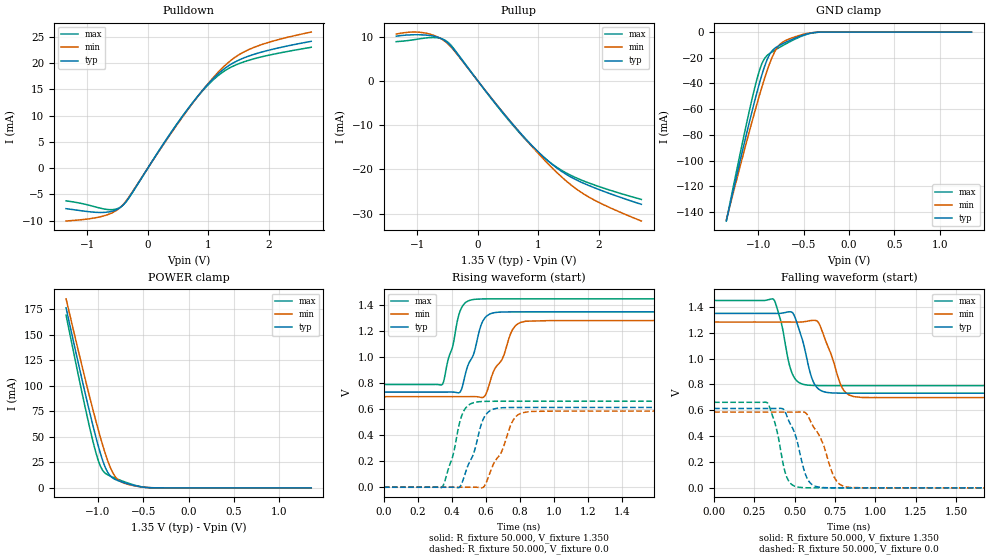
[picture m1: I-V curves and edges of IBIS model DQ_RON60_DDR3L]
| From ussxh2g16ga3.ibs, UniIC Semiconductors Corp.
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|   Model DQ_RON60_DDR3L
[Model] DQ_RON60_DDR3L
Model_type I/O
Vinl =  0.540V
Vinh =  0.810V
Vmeas =  0.675V
Rref =  50.000
Vref =  0.675V
C_comp   0.966pF   0.965pF   0.967pF
[Model Spec]
Vinh   0.810V   0.776V   0.860V
Vinl   0.540V   0.506V   0.590V
Vmeas   0.675V   0.641V   0.725V
Vref   0.675V   0.641V   0.725V
Rref   50.000   NA   NA
[Temperature Range]   25.000   95.000   -40.000
[Voltage Range]   1.350V   1.283V   1.450V
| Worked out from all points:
|   slope of the pulldown table from 0 to 0.203 V, typ, clamps not added: 55.8 ohm
|   slope of the pullup table from 0 to 0.203 V, typ, clamps not added: 56.9 ohm
|   GND clamp passes 1 mA (typ) near -0.43 V on its own axis
|   POWER clamp passes 1 mA (typ) near -0.52 V on its own axis
|   rising waveform, R_fixture 50.000, V_fixture 1.350: 20-80 % time 89.6ps typ, 116ps min, 71.1ps max; typ from 0.732 V to 1.35 V
|   rising waveform, R_fixture 50.000, V_fixture 0.0: 20-80 % time 92.1ps typ, 117ps min, 75ps max; typ from 0 V to 0.614 V
|   falling waveform, R_fixture 50.000, V_fixture 1.350: 20-80 % time 77.6ps typ, 95.9ps min, 66ps max; typ from 1.35 V to 0.732 V
|   falling waveform, R_fixture 50.000, V_fixture 0.0: 20-80 % time 87.7ps typ, 115ps min, 67.6ps max; typ from 0.614 V to 0 V
[Pulldown]
|Voltage   I(typ)   I(min)   I(max)
-1.35V    -7.722mA   -10.07mA   -6.234mA
-735mV    -8.434mA   -9.119mA   -7.75mA
-571mV    -8.147mA   -8.411mA   -7.895mA
-448mV    -7.434mA   -7.423mA   -7.4mA
-325mV    -5.846mA   -5.707mA   -5.893mA
249mV     4.444mA    4.346mA    4.482mA
618mV     10.59mA    10.47mA    10.61mA
905mV     14.83mA    14.84mA    14.73mA
1.151V    17.85mA    18.14mA    17.54mA
1.397V    19.96mA    20.76mA    19.37mA
1.684V    21.43mA    22.68mA    20.61mA
2.7V      24.18mA    25.94mA    23.04mA
[Pullup]
|Voltage   I(typ)   I(min)   I(max)
-1.35V    10.13mA    10.63mA    8.905mA
-908mV    10.43mA    10.94mA    9.653mA
-703mV    10.05mA    10.19mA    9.819mA
-539mV    9.062mA    8.911mA    9.199mA
-416mV    7.422mA    7.241mA    7.626mA
568mV     -9.667mA   -9.643mA   -9.848mA
855mV     -14.05mA   -14.22mA   -14.21mA
1.142V    -17.88mA   -18.48mA   -17.87mA
1.429V    -20.86mA   -22.25mA   -20.57mA
1.757V    -23.19mA   -25.63mA   -22.66mA
2.126V    -25.2mA    -28.3mA    -24.45mA
2.7V      -27.89mA   -31.66mA   -26.78mA
[GND_clamp]
|Voltage   I(typ)   I(min)   I(max)
-1.35V    -146.9mA   -146.3mA   -147.1mA
-1.126V   -78.8mA    -85.17mA   -70.77mA
-1.014V   -47.25mA   -56.31mA   -36.92mA
-958mV    -33.17mA   -42.77mA   -24.44mA
-930mV    -26.97mA   -36.36mA   -20.61mA
-874mV    -17.51mA   -24.69mA   -16.72mA
-818mV    -12.71mA   -15.46mA   -14.21mA
-762mV    -10.26mA   -9.751mA   -11.88mA
-706mV    -8.307mA   -6.907mA   -9.644mA
-538mV    -3.274mA   -2.499mA   -3.731mA
-398mV    -591.2uA   -439.3uA   -663.7uA
1.35V     0A         0A         0A
[POWER_clamp]
|Voltage   I(typ)   I(min)   I(max)
-1.35V    176.6mA    185.4mA    169.4mA
-1.198V   115.5mA    128.2mA    103.2mA
-1.114V   83.04mA    97.6mA     68.48mA
-1.058V   62.42mA    77.92mA    46.98mA
-1.002V   43.19mA    59.09mA    28.56mA
-946mV    26.54mA    41.57mA    16.92mA
-890mV    14.85mA    26.22mA    12.66mA
-834mV    9.439mA    14.55mA    10.39mA
-778mV    7.089mA    7.901mA    8.361mA
-638mV    3.198mA    2.764mA    3.815mA
-414mV    126.6uA    165.9uA    94.28uA
1.35V     0A         0A         0A
[Ramp]
| variable   typ   min   max
dV/dt_r   0.369/92.016p   0.352/0.117n   0.397/75.241p
dV/dt_f   0.371/77.557p   0.351/96.063p   0.395/65.845p
R_load = 50.000
[Rising Waveform]
R_fixture= 50.000
V_fixture= 1.350
V_fixture_min= 1.283
V_fixture_max= 1.450
|time   V(typ)   V(min)   V(max)
0s        732.3mV    697.2mV    791mV
345ps     732.3mV    697.2mV    794.6mV
448ps     734.1mV    697.2mV    1.359V
493ps     937.5mV    697.3mV    1.433V
521ps     1.006V     697.7mV    1.444V
566ps     1.231V     692.5mV    1.449V
602ps     1.316V     725.9mV    1.45V
756ps     1.35V      1.215V     1.45V
834ps     1.35V      1.278V     1.45V
3ns       1.35V      1.283V     1.45V
[Rising Waveform]
R_fixture= 50.000
V_fixture= 0.0
V_fixture_min= 0.0
V_fixture_max= 0.0
|time   V(typ)   V(min)   V(max)
0s        169.2nV    1.221uV    70.74nV
342ps     -22.87uV   2.873uV    391.3uV
403ps     351.9uV    3.439uV    233.7mV
457ps     29.71mV    -21.48uV   551.7mV
544ps     340.8mV    -48.08uV   655.9mV
577ps     504.3mV    -4.098mV   659.9mV
616ps     582.5mV    87.28mV    661.4mV
751ps     613.9mV    498mV      662mV
811ps     614.2mV    573mV      662mV
3ns       614.2mV    586.3mV    662mV
[Falling Waveform]
R_fixture= 50.000
V_fixture= 1.350
V_fixture_min= 1.283
V_fixture_max= 1.450
|time   V(typ)   V(min)   V(max)
0s        1.35V      1.283V     1.45V
370ps     1.35V      1.283V     1.457V
417ps     1.351V     1.283V     1.276V
483ps     1.359V     1.283V     888.3mV
569ps     1.037V     1.288V     797mV
607ps     845.8mV    1.296V     792.7mV
646ps     766.8mV    1.281V     791.4mV
796ps     732.6mV    769.9mV    791mV
867ps     732.3mV    705.8mV    791mV
3ns       732.3mV    697.2mV    791mV
[Falling Waveform]
R_fixture= 50.000
V_fixture= 0.0
V_fixture_min= 0.0
V_fixture_max= 0.0
|time   V(typ)   V(min)   V(max)
0s        614.2mV    586.3mV    662mV
332ps     614.2mV    586.3mV    656.2mV
385ps     614.2mV    586.3mV    465.3mV
447ps     570.2mV    586.3mV    94.63mV
518ps     346.9mV    586.4mV    6.391mV
595ps     39.21mV    523.5mV    351.2uV
674ps     2.358mV    346.2mV    15.86uV
741ps     209.2uV    90.6mV     1.342uV
818ps     12.47uV    7.593mV    273.5nV
3ns       174.2nV    1.214uV    191.5nV
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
